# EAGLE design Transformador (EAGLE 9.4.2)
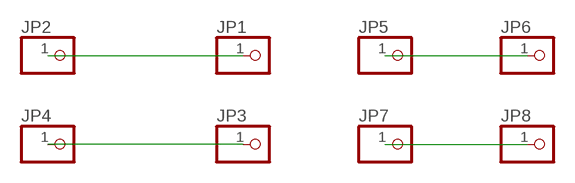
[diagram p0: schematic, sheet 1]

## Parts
JP1  PINHD-1X1  [1X01]
JP2  PINHD-1X1  [1X01]
JP3  PINHD-1X1  [1X01]
JP4  PINHD-1X1  [1X01]
JP5  PINHD-1X1  [1X01]
JP6  PINHD-1X1  [1X01]
JP7  PINHD-1X1  [1X01]
JP8  PINHD-1X1  [1X01]

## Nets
N$1: JP1.1 JP2.1
N$2: JP3.1 JP4.1
N$3: JP5.1 JP6.1
N$4: JP7.1 JP8.1

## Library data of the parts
JP1-JP8 = pinhead:PINHD-1X1: PIN HEADER

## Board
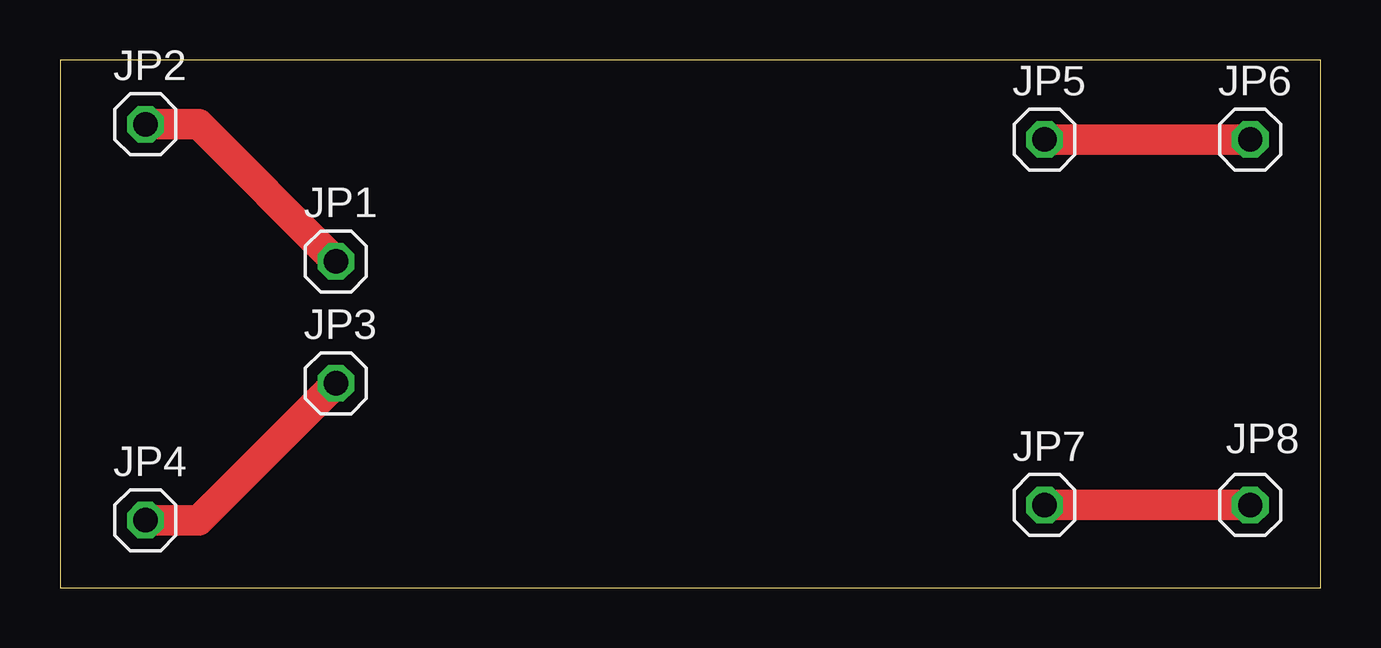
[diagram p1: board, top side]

Size 52.54 x 22 mm. Coordinates in mm from the lower left corner, seen from the top.
Outline: 52.54,22 0,22 0,0 52.54,0 52.54,22
Copper layers (1*16): Top 0.035mm / dielectric 1.5mm / Bottom 0.035mm
Design rules "default": minimum track width 6mil, minimum drill 0.35mm, track to track 6mil, track to pad 6mil, pad to pad 6mil, via to via 6mil, smd to smd 6mil, copper to edge 40mil, drill to drill 6mil, minimum pad ring 10mil, minimum via ring 8mil, stop-mask expansion 4mil, vias tented up to drill 0mil, thermal gap 10mil

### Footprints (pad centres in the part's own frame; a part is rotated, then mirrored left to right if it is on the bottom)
1X01 = drill 1.016 octagon: 1 0,0

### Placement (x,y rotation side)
JP1  11.49,13.6 0 top
JP2  3.55,19.31 0 top
JP3  11.49,8.52 0 top
JP4  3.55,2.81 0 top
JP5  41.02,18.68 0 top
JP6  49.59,18.68 0 top
JP7  41.02,3.44 0 top
JP8  49.59,3.44 0 top

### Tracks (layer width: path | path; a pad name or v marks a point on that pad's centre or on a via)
N$1
  Top 1.27: JP2.1 5.78,19.31 JP1.1
N$2
  Top 1.27: JP4.1 5.78,2.81 JP3.1
N$3
  Top 1.27: JP5.1 JP6.1
N$4
  Top 1.27: JP7.1 JP8.1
